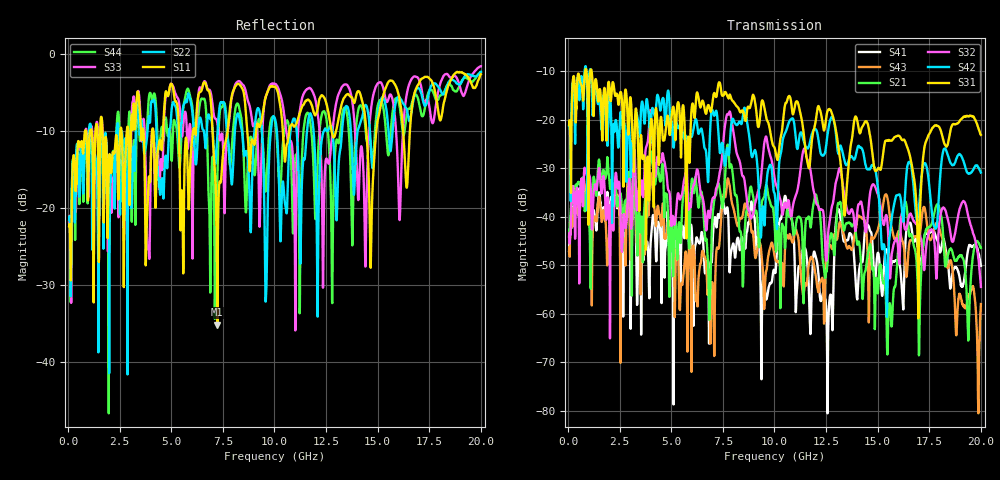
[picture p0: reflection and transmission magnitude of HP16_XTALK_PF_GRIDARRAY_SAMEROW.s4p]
# MHz S MA R 50.00
! FREQ  S11  S12  S13  S14
!  S21  S22  S23  S24
!  S31  S32  S33  S34
!  S41  S42  S43  S44
!  MAG  ANG  MAG  ANG  MAG  ANG  MAG  ANG
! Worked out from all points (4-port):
!   1996 points, 50 MHz to 20 GHz, reference 50 ohm
!   strongest paths, dB at 50 MHz, 5.04 GHz, 10.03 GHz, 15.02 GHz, 20 GHz:
!     S31: -21.2, -18.3, -26.2, -30.0, -23.2
!     S42: -21.3, -20.6, -35.9, -34.3, -30.9
!     S32: -44.1, -40.7, -32.7, -35.5, -54.5
!     S21: -43.9, -43.5, -43.6, -55.3, -46.4
!     S43: -47.1, -43.6, -48.6, -42.5, -58.0
!     S41: -47.1, -44.3, -51.6, -47.4, -50.1
!   lowest |S11| = -35.2 dB at 7.23 GHz (marker M1), VSWR 1.04, Z = 51.3 - j1.17 ohm
!   |S11| at or under -10 dB: start of sweep to 821.9 MHz; 1.666 GHz to 2.532 GHz (866 MHz wide, 41.3 % of centre); 6.999 GHz to 7.726 GHz (727 MHz wide, 9.87 % of centre)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
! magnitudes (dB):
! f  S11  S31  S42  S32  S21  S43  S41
! 50 MHz  -22.4  -21.2  -21.3  -44.1  -43.9  -47.1  -47.1
! 7.23 GHz  -35.2  -14.2  -19.6  -33.7  -33.7  -46.5  -40.7
! 12.8 GHz  -10.4  -19.0  -19.4  -37.6  -44.2  -46.6  -62.8
! 15.43 GHz  -4.1  -24.3  -57.9  -39.8  -61.5  -35.5  -46.8
! 16.33 GHz  -14.5  -24.5  -35.2  -42.7  -36.9  -49.2  -46.5
! 16.97 GHz  -3.9  -61.0  -39.6  -42.5  -59.9  -44.6  -47.0
! 20 GHz  -2.6  -23.2  -30.9  -54.5  -46.4  -58.0  -50.1
